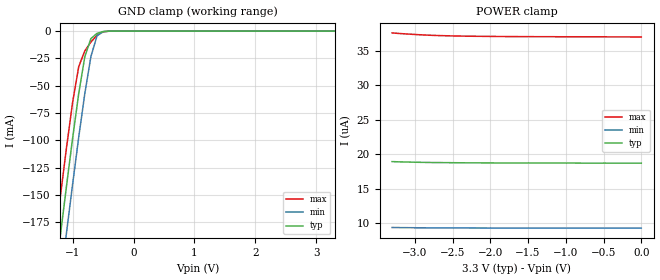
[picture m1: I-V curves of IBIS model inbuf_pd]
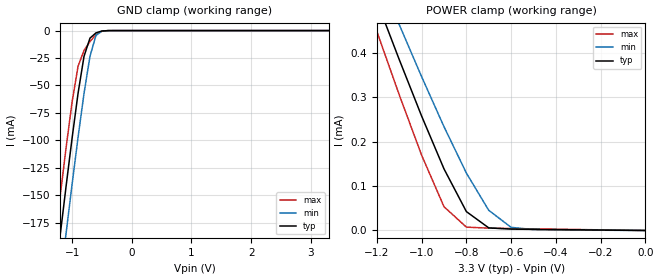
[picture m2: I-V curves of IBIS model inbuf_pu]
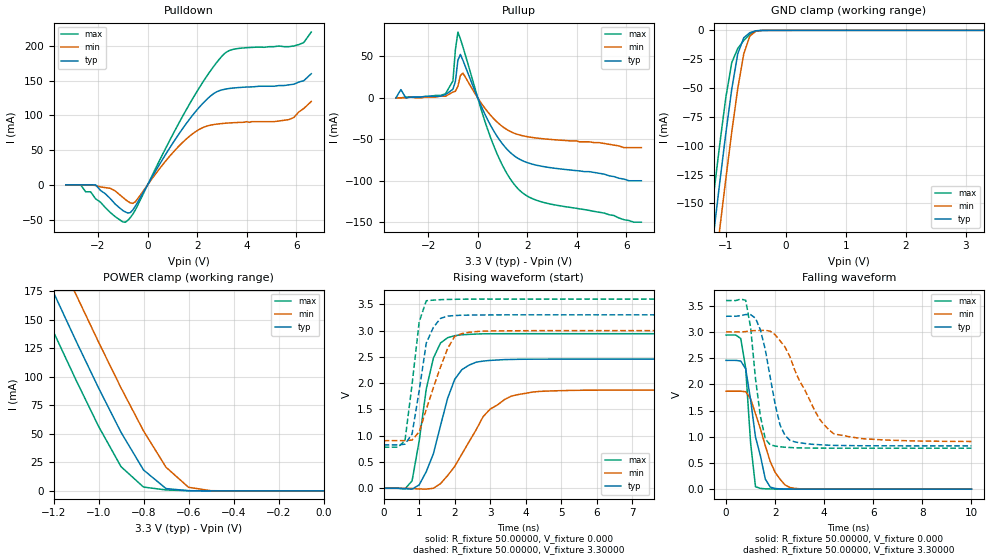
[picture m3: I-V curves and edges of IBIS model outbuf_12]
| IBIS file idt23s09_12.ibs created by s2ibis2 version 1.2
| North Carolina State University Electronics Research Laboratory  1995
[IBIS ver]   2.1
[File name]   idt23s09_12.ibs
[File Rev]   2.1
[Date]   Thursday, August 25 , 2005
[Source]   IDT
[Notes]   1. Temp typ=25C, min=-40C, max=100C
   2. IDT 0.5 process
   3. Ramp rates based on 50 ohm load
[Disclaimer]
Integrated Device Technology, Inc. ("IDT") hereby grants the user of this
IBIS model ("User") a non-exclusive, nontransferable license to use this
IBIS model under the following terms: The User is granted this license only
to use the IBIS model for demonstration purposes only and is not granted
rights to sell, copy (except as needed to run the IBIS model), rent, lease
or sub-license (except for demonstration) the IBIS model in whole or in
part, or in modified form to anyone. The User may modify the IBIS model to
suit its specific applications, but  rights to derivative works and such
modifications shall belong to IDT.
THIS IBIS MODEL IS PROVIDED ON AN AS IS" BASIS AND IDT  MAKES ABSOLUTELY NO
WARRANTY WITH RESPECT TO THE INFORMATION CONTAINED HEREIN.  IDT DISCLAIMS
AND USER WAIVES ALL WARRANTIES, EXPRESS AND IMPLIED, INCLUDING WARRANTIES OF
MERCHANTABILITY AND FITNESS FOR A PARTICULAR PURPOSE.  THE ENTIRE RISK AS TO
QUALITY AND PERFORMANCE IS WITH THE USER  ACCORDINGLY, IN NO EVENT SHALL IDT
BE LIABLE FOR ANY DIRECT OR INDIRECT DAMAGES, WHETHER IN CONTRACT OR TORT,
INCLUDING ANY LOST PROFITS OR OTHER INCIDENTAL, CONSEQUENTIAL, EXEMPLARY, OR
PUNITIVE DAMAGES ARISING OUT OF THE USE OR APPLICATION OF THE  IBIS MODEL,
WHETHER OR NOT IDT HAD NOTICE OF SUCH DAMAGES.
IDT reserves the right to make changes without notice to any product herein
to improve reliability, function, or design. IDT does not convey any license
under patent rights or any other intellectual property rights, including
those of third parties. IDT is not obligated to provide maintenance or
support for the licensed IBIS model.
*This model is for the 3.3V Zero Delay Clock Buffer, Spread Spectrum
*Compatible
[Copyright]
Copyright 2002, Integrated Device Technology, Inc. All rights reserved.
|History
|Rev 1.0 Created on October 21 2003
|   2.0 Regenerated file on August 18 2005
|   2.1 GND and POWER clamp current with a 2ohm resistor in series with
|   pin to simulate diode resistance August 25 2005
|   Component IDT23S09-1H
[Component]   IDT23S09-1H
[Manufacturer]   Integrated Device Technology, Inc.
[Package]
|SO16-10 (Thin Shrink Size Outline Package)
| variable   typ   min   max
R_pkg   52.59m   52.19m   52.96m
L_pkg   4.36nH   3.91nH   4.78nH
C_pkg   0.24pF   0.22pF   0.29pF
|SO16-8 (Small Outline Package)
|[R_pkg]   53.14m   52.77m   53.55m
|[L_pkg]   5.18nH   4.04nH   6.38nH
|[C_pkg]   0.38pF   0.224pF   0.551pF
[Pin]  signal_name   model_name   R_pin   L_pin   C_pin
1   REF   inbuf_pd
2   CLKA1   outbuf_12
3   CLKA2   outbuf_12
4   VDD   POWER
5   GND   GND
6   CLKB1   outbuf_12
7   CLKB2   outbuf_12
8   S2   inbuf_pu
9   S1   inbuf_pu
10   CLKA1   outbuf_12
11   CLKA2   outbuf_12
12   GND   GND
13   VDD   POWER
14   CLKA1   outbuf_12
15   CLKA2   outbuf_12
16   CLKOUT   outbuf_12
| Models and submodels in the file (3): inbuf_pd (Input), inbuf_pu (Input), outbuf_12 (3-state)
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| d   d   dummy_model
| oe   oe   dummy_model
|   Model inbuf_pd
[Model]   inbuf_pd
Model_type   Input
Vinl =  0.80000V
Vinh =  2.00000V
C_comp   5.25000pF   5.25000pF   5.25000pF
[Temperature Range]   25.00000   100.00000   -40.00000
[Voltage Range]   3.30000V   3.00000V   3.60000V
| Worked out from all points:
|   GND clamp passes 1 mA (typ) near -0.54 V on its own axis
[GND_clamp]
| voltage   I(typ)   I(min)   I(max)
-3.3V     -1.185A    -1.225A    -1.151A
-1.3V     -232.4mA   -275.4mA   -196.4mA
-1.2V     -186.6mA   -229.6mA   -150.8mA
-1.1V     -141.6mA   -184.4mA   -106.5mA
-1V       -98mA      -140.1mA   -65.13mA
-900mV    -57.16mA   -97.22mA   -32.53mA
-800mV    -23.43mA   -57.16mA   -18.11mA
-700mV    -6.867mA   -23.35mA   -9.97mA
-600mV    -2.108mA   -4.373mA   -3.788mA
-500mV    -376.3uA   -455.1uA   -637.4uA
-400mV    -39.97uA   -43.59uA   -54.23uA
3.3V      18.7uA     9.282uA    36.99uA
[POWER_clamp]
| voltage   I(typ)   I(min)   I(max)
-3.3V     18.93uA    9.375uA    37.59uA
-3.2V     18.89uA    9.361uA    37.5uA
-3V       18.84uA    9.34uA     37.36uA
-2.8V     18.8uA     9.325uA    37.25uA
-2.5V     18.77uA    9.311uA    37.15uA
-2.3V     18.75uA    9.305uA    37.11uA
-1.8V     18.73uA    9.297uA    37.06uA
-1.5V     18.73uA    9.293uA    37.05uA
-1.4V     18.72uA    9.292uA    37.04uA
-900mV    18.72uA    9.288uA    37.03uA
-800mV    18.71uA    9.287uA    37.03uA
0V        18.7uA     9.279uA    37uA
|   Model inbuf_pu
[Model]   inbuf_pu
Model_type   Input
Vinl =  0.80000V
Vinh =  2.00000V
C_comp   5.25000pF   5.25000pF   5.25000pF
[Temperature Range]   25.00000   100.00000   -40.00000
[Voltage Range]   3.30000V   3.00000V   3.60000V
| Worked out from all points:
|   GND clamp passes 1 mA (typ) near -0.54 V on its own axis
|   POWER clamp passes 1 mA (typ) near -1.56 V on its own axis
[GND_clamp]
| voltage   I(typ)   I(min)   I(max)
-3.3V     -1.185A    -1.225A    -1.151A
-1.3V     -232.4mA   -275.4mA   -196.4mA
-1.2V     -186.6mA   -229.6mA   -150.8mA
-1.1V     -141.6mA   -184.4mA   -106.5mA
-1V       -98mA      -140.1mA   -65.13mA
-900mV    -57.16mA   -97.22mA   -32.53mA
-800mV    -23.43mA   -57.16mA   -18.11mA
-700mV    -6.865mA   -23.35mA   -9.967mA
-600mV    -2.105mA   -4.372mA   -3.785mA
-500mV    -373.2uA   -453.1uA   -633.1uA
-400mV    -37.63uA   -42.04uA   -50.7uA
3.3V      26pA       932.9nA    -1.919uA
[POWER_clamp]
| voltage   I(typ)   I(min)   I(max)
-3.3V     3.436mA    3.233mA    3.639mA
-1.3V     650.7uA    705.6uA    594.8uA
-1.2V     516.8uA    584uA      448.6uA
-1.1V     385.3uA    464.1uA    305.8uA
-1V       257.9uA    346.7uA    169.7uA
-900mV    138.8uA    233.9uA    53.5uA
-800mV    42.53uA    129.4uA    7.547uA
-700mV    5.822uA    45.39uA    5.256uA
-600mV    3.108uA    7.059uA    4.42uA
-500mV    2.493uA    1.92uA     3.634uA
0V        25.99pA    392.8pA    1.378pA
|   Model outbuf_12
[Model]   outbuf_12
Model_type   3-state
Polarity   Non-Inverting
Enable   Active-High
Vmeas =  1.650000V
C_comp   7.00000pF   7.00000pF   7.00000pF
[Temperature Range]   25.00000   100.00000   -40.00000
[Voltage Range]   3.30000V   3.00000V   3.60000V
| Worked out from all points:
|   slope of the pulldown table from 0 to 0.495 V, typ, clamps not added: 16.3 ohm
|   slope of the pullup table from 0 to 0.495 V, typ, clamps not added: 15.5 ohm
|   GND clamp passes 1 mA (typ) near -0.54 V on its own axis
|   POWER clamp passes 1 mA (typ) near -0.64 V on its own axis
|   rising waveform, R_fixture 50.00000, V_fixture 0.000: 20-80 % time 639ps typ, 1.03ns min, 440ps max; typ from 0 V to 2.46 V
|   rising waveform, R_fixture 50.00000, V_fixture 3.30000: 20-80 % time 358ps typ, 638ps min, 296ps max; typ from 0.826 V to 3.3 V
|   falling waveform, R_fixture 50.00000, V_fixture 0.000: 20-80 % time 554ps typ, 789ps min, 287ps max; typ from 2.46 V to 0 V
|   falling waveform, R_fixture 50.00000, V_fixture 3.30000: 20-80 % time 628ps typ, 1.28ns min, 410ps max; typ from 3.3 V to 0.826 V
[Pulldown]
| voltage   I(typ)   I(min)   I(max)
-3.3V     0A         0A         0A
-2.7V     0A         0A         0A
-2.1V     0A         -1mA       -20mA
-900mV    -38.9mA    -21mA      -53.78mA
-500mV    -30.94mA   -24.53mA   -36.5mA
800mV     48.01mA    37.38mA    57.64mA
1.8V      99.54mA    73.1mA     123.1mA
3V        136.8mA    88.31mA    185.5mA
3.6V      139.9mA    89.75mA    196.2mA
5.7V      144mA      94mA       199mA
6.3V      150mA      110mA      205mA
6.6V      160mA      120mA      220mA
[Pullup]
| voltage   I(typ)   I(min)   I(max)
-3.3V     0A         0A         0A
-3.1V     10mA       0A         0A
-2.9V     0A         0A         1mA
-1.3V     4mA        2mA        5mA
-1V       10.4mA     7mA        20.5mA
-900mV    20.1mA     8mA        58.5mA
-800mV    45.49mA    14mA       79.4mA
-600mV    45.55mA    29.88mA    61.76mA
600mV     -37.56mA   -23.69mA   -54.38mA
1.6V      -72.51mA   -44.01mA   -108.8mA
2.6V      -82.61mA   -49.21mA   -125.7mA
6.6V      -100mA     -60mA      -150mA
[GND_clamp]
| voltage   I(typ)   I(min)   I(max)
-3.3V     -1.149A    -1.186A    -1.117A
-1.3V     -219.9mA   -260.2mA   -186mA
-1.2V     -175.4mA   -215.8mA   -141.6mA
-1.1V     -131.7mA   -171.9mA   -98.54mA
-1V       -89.63mA   -129.1mA   -58.47mA
-900mV    -50.73mA   -88.06mA   -27.87mA
-800mV    -20.23mA   -50.36mA   -15.65mA
-700mV    -6.448mA   -20.37mA   -8.749mA
-600mV    -2.008mA   -5.028mA   -3.424mA
-500mV    -368.8uA   -702.4uA   -604.5uA
-400mV    -39.53uA   -59.24uA   -52.53uA
3.3V      18.42uA    10.23uA    36.55uA
[POWER_clamp]
| voltage   I(typ)   I(min)   I(max)
-3.3V     1.109A     1.147A     1.078A
-1.3V     216.7mA    257.2mA    182.3mA
-1.2V     173.7mA    214.3mA    139.2mA
-1.1V     131.3mA    171.9mA    97.06mA
-1V       90.24mA    130.4mA    56.63mA
-900mV    51.34mA    90.22mA    21.24mA
-800mV    18.35mA    52.57mA    3.384mA
-700mV    2.067mA    20.75mA    862.6uA
-600mV    211.3uA    3.195mA    172.4uA
-500mV    44.27uA    214.9uA    51.86uA
0V        18.42uA    9.13uA     36.56uA
[Ramp]
| variable   typ   min   max
dV/dt_r   1.47420/0.59066n   1.12140/1.07063n   1.76400/0.36489n
dV/dt_f   1.48392/0.59911n   1.25358/1.26920n   1.69050/0.34135n
R_load = 50.00000
[Rising Waveform]
R_fixture = 50.00000
V_fixture = 0.000
V_fixture_min = 0.000
V_fixture_max = 0.000
| time   V(typ)   V(min)   V(max)
0s        0V         0V         0V
800ps     -16.73mV   -4.785mV   141.3mV
1.2ns     317.4mV    -15.4mV    1.891V
1.4ns     656.1mV    285uV      2.475V
1.8ns     1.71V      241.1mV    2.864V
2ns       2.072V     415.7mV    2.902V
2.4ns     2.341V     880.3mV    2.927V
2.8ns     2.42V      1.363V     2.938V
3.6ns     2.45V      1.754V     2.94V
10ns      2.457V     1.869V     2.94V
[Rising Waveform]
R_fixture = 50.00000
V_fixture = 3.30000
V_fixture_min = 3.00000
V_fixture_max = 3.60000
| time   V(typ)   V(min)   V(max)
0s        825.8mV    906.5mV    781.4mV
600ps     838.8mV    906.5mV    904mV
800ps     1.032V     916.1mV    1.976V
1ns       1.854V     1.073V     3.165V
1.2ns     2.763V     1.499V     3.567V
1.4ns     3.061V     1.916V     3.579V
1.8ns     3.276V     2.659V     3.592V
2ns       3.285V     2.889V     3.595V
2.2ns     3.292V     2.942V     3.596V
10ns      3.299V     2.999V     3.599V
[Falling Waveform]
R_fixture = 50.00000
V_fixture = 0.000
V_fixture_min = 0.000
V_fixture_max = 0.000
| time   V(typ)   V(min)   V(max)
0s        2.457V     1.869V     2.94V
600ps     2.444V     1.869V     2.874V
800ps     2.297V     1.859V     2.307V
1ns       1.704V     1.723V     884.6mV
1.2ns     994.5mV    1.438V     47.53mV
1.6ns     192.3mV    827.3mV    6.553mV
1.8ns     39.98mV    528.3mV    3.956mV
2.2ns     4.999mV    190.6mV    2.12mV
2.6ns     3.043mV    32.54mV    1.147mV
10ns      -5.436uV   76.97uV    1.024uV
[Falling Waveform]
R_fixture = 50.00000
V_fixture = 3.30000
V_fixture_min = 3.00000
V_fixture_max = 3.60000
| time   V(typ)   V(min)   V(max)
0s        3.299V     2.999V     3.599V
800ps     3.331V     3.006V     3.604V
1ns       3.329V     3.019V     3.087V
1.4ns     3.038V     3.029V     1.389V
1.8ns     2.134V     3.014V     845.1mV
2.2ns     1.224V     2.832V     807.9mV
2.4ns     1.029V     2.712V     800mV
3.8ns     848mV      1.342V     782.8mV
4.4ns     835.3mV    1.053V     781.9mV
10ns      825.8mV    909.7mV    781.5mV
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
